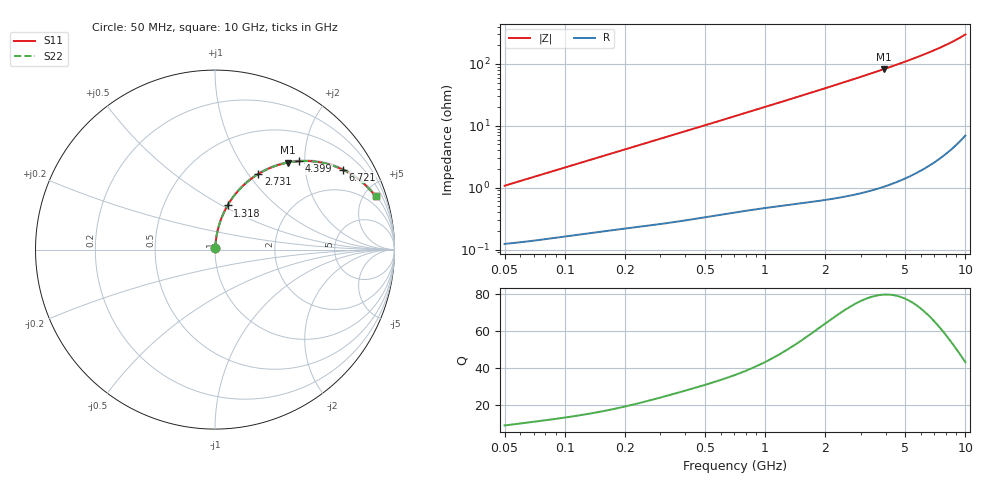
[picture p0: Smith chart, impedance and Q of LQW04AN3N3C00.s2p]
!Murata Part Number: LQW04AN3N3C00
!These Parameters are Measured in Series Mode Connection
!  o--[Z]--o
!Port1  Port2
!  o-------o
!Freq. Start=50[MHz] Stop=10[GHz], 401[Steps]
# Hz S RI R 50
!Freq.(Hz)	S 11(Real)	S 11(Imag)	S 21(Real)	S 21(Imag)	S 12(Real)	S 12(Imag)	S 22(Real)	S 22(Imag)
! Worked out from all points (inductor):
!   401 points, 50 MHz to 10 GHz, reference 50 ohm
!   read as one part in series: L = 3.38 nH near 51.34 MHz
!   highest Q = 79.8 at 3.905 GHz (marker M1), where L = 3.35 nH
!   S11 on the Smith chart (normalised r, x): 50 MHz: 1.00, +0.02; 1.318 GHz: 1.01, +0.53; 2.731 GHz: 1.02, +1.12; 4.399 GHz: 1.02, +1.88; 6.721 GHz: 1.05, +3.16; 10 GHz: 1.14, +6.00
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5e7  0.00134 0.0107  0.9987 -0.0107  0.9987 -0.0107  0.00134 0.0107
1.214486e8  0.00241 0.0253  0.9976 -0.0253  0.9976 -0.0253  0.00241 0.0253
1.956524e8  0.00377 0.0402  0.9962 -0.0402  0.9962 -0.0402  0.00377 0.0402
2.949953e8  0.00618 0.06  0.9938 -0.06  0.9938 -0.06  0.00618 0.06
4.689809e8  0.0122 0.0941  0.9878 -0.0941  0.9878 -0.0941  0.0122 0.0941
7.071068e8  0.0239 0.1394  0.9761 -0.1394  0.9761 -0.1394  0.0239 0.1394
9.717327e8  0.0413 0.1875  0.9587 -0.1875  0.9587 -0.1875  0.0413 0.1875
1.31782e9  0.0705 0.2462  0.9295 -0.2462  0.9295 -0.2462  0.0705 0.2462
1.717543e9  0.112 0.307  0.888 -0.307  0.888 -0.307  0.112 0.307
2.179987e9  0.1681 0.3666  0.8319 -0.3666  0.8319 -0.3666  0.1681 0.3666
2.730534e9  0.2419 0.4215  0.7581 -0.4215  0.7581 -0.4215  0.2419 0.4215
3.243629e9  0.3135 0.4575  0.6865 -0.4575  0.6865 -0.4575  0.3135 0.4575
3.904516e9  0.4047 0.4846  0.5953 -0.4846  0.5953 -0.4846  0.4047 0.4846
4.171863e9  0.4402 0.4902  0.5598 -0.4902  0.5598 -0.4902  0.4402 0.4902
4.398862e9  0.4695 0.4928  0.5305 -0.4928  0.5305 -0.4928  0.4695 0.4928
4.890587e9  0.5298 0.4927  0.4702 -0.4927  0.4702 -0.4927  0.5298 0.4927
5.437278e9  0.5912 0.485  0.4088 -0.485  0.4088 -0.485  0.5912 0.485
6.045081e9  0.6523 0.4693  0.3477 -0.4693  0.3477 -0.4693  0.6523 0.4693
6.720828e9  0.7115 0.4457  0.2885 -0.4457  0.2885 -0.4457  0.7115 0.4457
8.198065e9  0.8125 0.3815  0.1875 -0.3815  0.1875 -0.3815  0.8125 0.3815
9.236013e9  0.8643 0.3323  0.1357 -0.3323  0.1357 -0.3323  0.8643 0.3323
1e10  0.8944 0.2959  0.1056 -0.2959  0.1056 -0.2959  0.8944 0.2959
